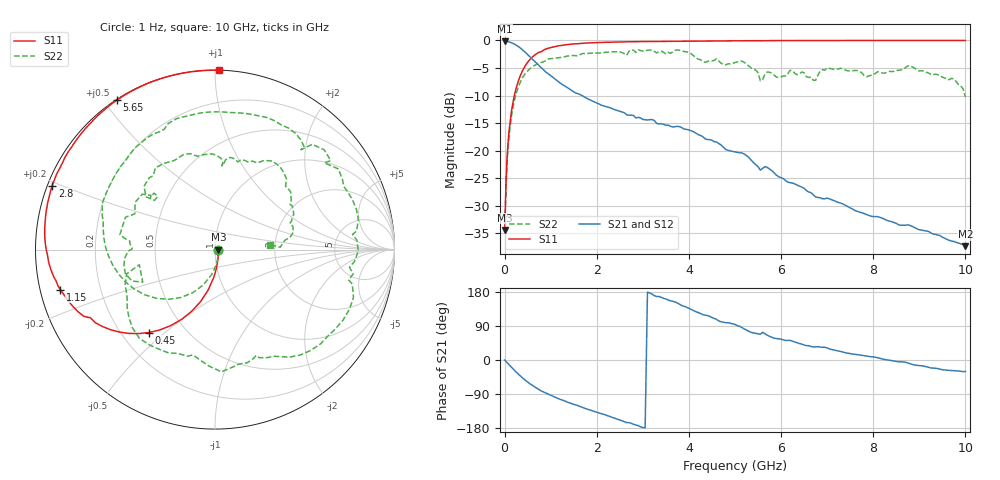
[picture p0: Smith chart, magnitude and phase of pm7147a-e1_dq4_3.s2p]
# GHz S DB R 50
! S-Parameters data
! Freq  dbS11  angS11  dbS21  angS21  dbS12  angS12  dbS22  angS22
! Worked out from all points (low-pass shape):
!   279 points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, 1 Hz to 10 GHz, reference 50 ohm
!   highest |S21| = -0.17 dB at 19.95 kHz (marker M1); lowest = -37.3 dB at 10 GHz (marker M2)
!   |S21| within 3 dB of the highest: start of sweep to 575.3 MHz
!   lowest |S11| = -34.4 dB at 19.95 kHz (marker M3), VSWR 1.04, Z = 51.9 - j0.0028 ohm
!   |S11| at or under -10 dB: start of sweep to 212.4 MHz
!   |S22| runs from -34.4 to -1.7 dB; largest |S21 - S12| = 0
!   S11 on the Smith chart (normalised r, x): 1 Hz: 1.04, -0.00; 450 MHz: 0.31, -0.44; 1.15 GHz: 0.06, -0.13; 2.8 GHz: 0.01, +0.19; 5.65 GHz: 0.00, +0.54; 10 GHz: 0.00, +1.02
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1e-09  -34.39 -0.0  -0.17 -0.0  -0.17 -0.0  -34.39 -0.0
1.99526e-05  -34.39 -0.1  -0.17 -0.0  -0.17 -0.0  -34.39 -0.1
0.06309573  -20.02 -84.9  -0.21 -8.2  -0.21 -8.2  -20.80 -87.8
0.15  -12.78 -99.7  -0.42 -19.3  -0.42 -19.3  -13.63 -108.4
0.45  -4.57 -128.5  -2.16 -53.5  -2.16 -53.5  -6.01 -153.9
0.75  -2.14 -148.6  -4.56 -78.2  -4.56 -78.2  -4.12 174.2
1.15  -1.00 -165.5  -7.39 -101.0  -7.39 -101.0  -3.14 142.0
1.7  -0.51 179.1  -10.10 -125.7  -10.10 -125.7  -2.37 106.1
2.3  -0.31 166.9  -12.25 -149.8  -12.25 -149.8  -2.04 68.5
2.8  -0.23 158.5  -13.62 -169.9  -13.62 -169.9  -1.79 37.5
3.35  -0.19 150.5  -15.16 167.5  -15.16 167.5  -2.02 3.7
3.75  -0.15 145.1  -15.59 150.5  -15.59 150.5  -1.73 -23.8
4.05  -0.13 141.3  -16.38 133.4  -16.38 133.4  -2.44 -51.1
5.05  -0.06 129.7  -20.32 90.7  -20.32 90.7  -3.92 -119.6
5.55  -0.03 124.3  -23.53 68.0  -23.53 68.0  -7.33 -168.7
5.65  -0.04 123.3  -22.90 69.2  -22.90 69.2  -6.12 -159.2
6.2  -0.02 117.8  -25.82 51.7  -25.82 51.7  -5.41 171.1
6.7  -0.01 113.1  -28.03 34.5  -28.03 34.5  -7.22 137.2
7.3  -0.01 107.9  -29.53 22.4  -29.53 22.4  -5.06 108.1
8.35  -0.00 99.6  -32.80 -0.4  -32.80 -0.4  -5.61 71.8
9.1  -0.00 94.4  -34.48 -16.3  -34.48 -16.3  -5.51 37.3
10  -0.00 88.6  -37.34 -30.2  -37.34 -30.2  -10.25 5.3
